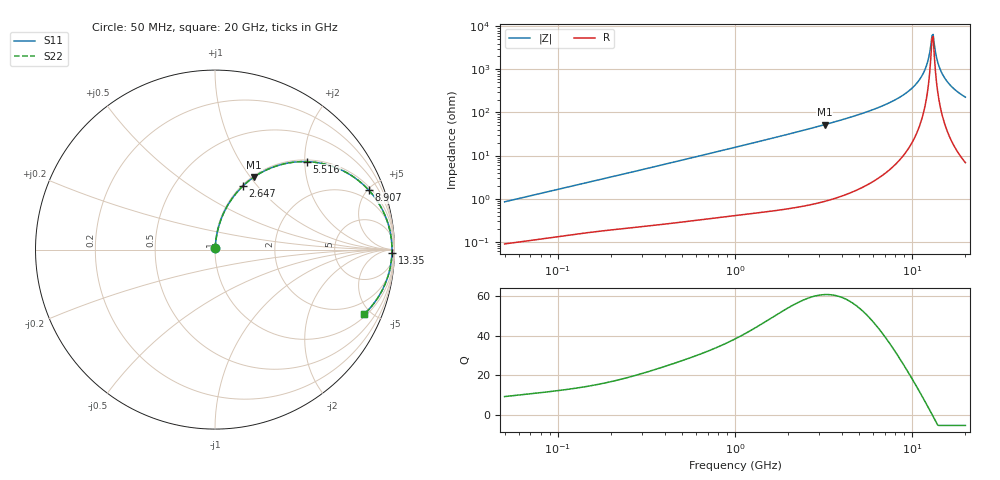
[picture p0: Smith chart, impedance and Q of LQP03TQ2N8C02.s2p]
!Murata Part Number: LQP03TQ2N8C02
!These Parameters are Measured in Series Mode Connection
!  o--[Z]--o
!Port1  Port2
!  o-------o
!Freq. Start=50[MHz] Stop=20[GHz], 401[Steps]
# Hz S RI R 50
!Freq.(Hz) S11(Real) S11(Imag) S21(Real) S21(Imag) S12(Real) S12(Imag) S22(Real) S22(Imag)
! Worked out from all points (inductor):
!   401 points, 50 MHz to 20 GHz, reference 50 ohm
!   read as one part in series: L = 2.64 nH near 51.52 MHz
!   highest Q = 60.5 at 3.217 GHz (marker M1), where L = 2.59 nH
!   self-resonance near 12.95 GHz
!   S11 on the Smith chart (normalised r, x): 50 MHz: 1.00, +0.02; 2.647 GHz: 1.01, +0.84; 5.516 GHz: 1.04, +2.05; 8.907 GHz: 1.20, +5.08; 13.35 GHz: 43, -65; 20 GHz: 1.14, -4.54
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5e7  0.000956 0.00837  0.999 -0.00837  0.999 -0.00837  0.000956 0.00837
1.364002e8  0.00204 0.0219  0.998 -0.0219  0.998 -0.0219  0.00204 0.0219
3.721004e8  0.00583 0.0578  0.9942 -0.0578  0.9942 -0.0578  0.00583 0.0578
1e9  0.0272 0.1502  0.9728 -0.1502  0.9728 -0.1502  0.0272 0.1502
2.647493e9  0.1555 0.354  0.8445 -0.354  0.8445 -0.354  0.1555 0.354
2.728004e9  0.164 0.362  0.836 -0.362  0.836 -0.362  0.164 0.362
3.216634e9  0.2189 0.4053  0.7811 -0.4053  0.7811 -0.4053  0.2189 0.4053
5.515528e9  0.5121 0.4901  0.4879 -0.4901  0.4879 -0.4901  0.5121 0.4901
7.442007e9  0.7332 0.4287  0.2668 -0.4287  0.2668 -0.4287  0.7332 0.4287
8.907419e9  0.8564 0.3318  0.1436 -0.3318  0.1436 -0.3318  0.8564 0.3318
1.019291e10  0.9286 0.23  0.0714 -0.23  0.0714 -0.23  0.9286 0.23
1.115139e10  0.9621 0.1511  0.0379 -0.1511  0.0379 -0.1511  0.9621 0.1511
1.201863e10  0.9794 0.0807  0.0206 -0.0807  0.0206 -0.0807  0.9794 0.0807
1.238412e10  0.9834 0.0519  0.0166 -0.0519  0.0166 -0.0519  0.9834 0.0519
1.276073e10  0.9857 0.0228  0.0143 -0.0228  0.0143 -0.0228  0.9857 0.0228
1.295331e10  0.9862 0.00818  0.0138 -0.00818  0.0138 -0.00818  0.9862 0.00818
1.334722e10  0.9858 -0.021  0.0142 0.021  0.0142 0.021  0.9858 -0.021
1.375312e10  0.9838 -0.0502  0.0162 0.0502  0.0162 0.0502  0.9838 -0.0502
1.417136e10  0.98 -0.0791  0.02 0.0791  0.02 0.0791  0.98 -0.0791
1.527346e10  0.9633 -0.1496  0.0367 0.1496  0.0367 0.1496  0.9633 -0.1496
1.721783e10  0.9165 -0.2537  0.0835 0.2537  0.0835 0.2537  0.9165 -0.2537
2e10  0.8302 -0.3607  0.1698 0.3607  0.1698 0.3607  0.8302 -0.3607
